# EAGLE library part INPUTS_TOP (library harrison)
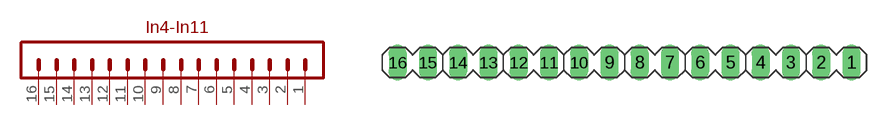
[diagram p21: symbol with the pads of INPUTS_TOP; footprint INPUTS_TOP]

Designator prefix -

## INPUTS_TOP  [INPUTS_TOP]
1  P$16  pas
2  P$15  pas
3  P$14  pas
4  P$13  pas
5  P$12  pas
6  P$11  pas
7  P$10  pas
8  P$9  pas
9  P$8  pas
10  P$7  pas
11  P$6  pas
12  P$5  pas
13  P$4  pas
14  P$3  pas
15  P$2  pas
16  P$1  pas

## Footprint INPUTS_TOP (pad centres in mm)
drill 1.016 long: 1 19.685,0; 2 17.145,0; 3 14.605,0; 4 12.065,0; 5 9.525,0; 6 6.985,0; 7 4.445,0; 8 1.905,0; 9 -0.635,0; 10 -3.175,0; 11 -5.715,0; 12 -8.255,0; 13 -10.795,0; 14 -13.335,0; 15 -15.875,0; 16 -18.415,0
